(* Logix 5000 AddOnInstructionDefinition export OM_AZ_MOVE; software revision 32.00 *)

ADD_ON_INSTRUCTION OM_AZ_MOVE   (* revision 1.3 U1.0, vendor ORIENTALMOTOR CO.,LTD. *)
// Revision note:
// Implicit message based on AZD-AEP,-CEP and -KEP.
// Help:
// This AOI is used to select and operate a pre-programmed data operation. This is used when the same operation is used repeatedly.
VAR_IN_OUT
   ImplicitMSGinput : INT[28]; {required}   // Implicit message Input (driver->scanner)
        [0]   // Remote I/O (R-OUT)
        [0].0   // R-OUT0
        [0].1   // R-OUT1
        [0].2   // R-OUT2
        [0].3   // R-OUT3
        [0].4   // R-OUT4
        [0].5   // R-OUT5
        [0].6   // R-OUT6
        [0].7   // R-OUT7
        [0].8   // R-OUT8
        [0].9   // R-OUT9
        [0].10   // R-OUT10
        [0].11   // R-OUT11
        [0].12   // R-OUT12
        [0].13   // R-OUT13
        [0].14   // R-OUT14
        [0].15   // R-OUT15
        [1]   // Operation data number selection_R
        [1].0   // M0_R
        [1].1   // M1_R
        [1].2   // M2_R
        [1].3   // M3_R
        [1].4   // M4_R
        [1].5   // M5_R
        [1].6   // M6_R
        [1].7   // M7_R
        [1].8   // Reserved
        [1].9   // Reserved
        [1].10   // Reserved
        [1].11   // Reserved
        [1].12   // Reserved
        [1].13   // Reserved
        [1].14   // Reserved
        [1].15   // Reserved
        [2]   // Fixed I/O (OUT)
        [2].0   // SEQ-BSY
        [2].1   // MOVE
        [2].2   // IN-POS
        [2].3   // START_R
        [2].4   // HOME-END
        [2].5   // READY
        [2].6   // DCMD-RDY
        [2].7   // ALM-A
        [2].8   // TRIG_R
        [2].9   // TRIG-MODE_R
        [2].10   // SET-ERR
        [2].11   // EXE-ERR
        [2].12   // DCMD-FULL
        [2].13   // STOP_R
        [2].14   // ETO-MON
        [2].15   // TLC
        [3]   // Present alarm
        [4]   // Feedback position (lower)
        [5]   // Feedback position (upper)
        [6]   // Feedback speed [Hz] (lower)
        [7]   // Feedback speed [Hz] (upper)
        [8]   // Command position (lower)
        [9]   // Command position (upper)
        [10]   // Torque monitor
        [11]   // CST operating current
        [12]   // Information (lower)
        [13]   // Information (upper)
        [14]   // Reserved
        [15]   // Read parameter ID_R
        [16]   // Read/write status
        [16].0   // Reserved
        [16].1   // Reserved
        [16].2   // Reserved
        [16].3   // Reserved
        [16].4   // Reserved
        [16].5   // Reserved
        [16].6   // Reserved
        [16].7   // RD-ERR
        [16].8   // WR-END
        [16].9   // SYS-BSY
        [16].10   // Reserved
        [16].11   // WR-SET-ERR
        [16].12   // WR-IF-ERR
        [16].13   // WR-NV-ERR
        [16].14   // WR-EXE-ERR
        [16].15   // WR-ERR
        [17]   // Write parameter ID_R
        [18]   // Read data (lower)
        [19]   // Read data (upper)
        [20]   // Assignable monitor 0 (lower)
        [21]   // Assignable monitor 0 (upper)
        [22]   // Assignable monitor 1 (lower)
        [23]   // Assignable monitor 1 (upper)
        [24]   // Assignable monitor 2 (lower)
        [25]   // Assignable monitor 2 (upper)
        [26]   // Assignable monitor 3 (lower)
        [27]   // Assignable monitor 3 (upper)
   ImplicitMSGoutput : INT[20]; {required}   // Implicit message Output (scanner->driver)
        [0]   // Remote I/O(R-IN)
        [0].0   // R-IN0
        [0].1   // R-IN1
        [0].2   // R-IN2
        [0].3   // R-IN3
        [0].4   // R-IN4
        [0].5   // R-IN5
        [0].6   // R-IN6
        [0].7   // R-IN7
        [0].8   // R-IN8
        [0].9   // R-IN9
        [0].10   // R-IN10
        [0].11   // R-IN11
        [0].12   // R-IN12
        [0].13   // R-IN13
        [0].14   // R-IN14
        [0].15   // R-IN15
        [1]   // Operation data number selection
        [1].0   // M0
        [1].1   // M1
        [1].2   // M2
        [1].3   // M3
        [1].4   // M4
        [1].5   // M5
        [1].6   // M6
        [1].7   // M7
        [1].8   // Reserved
        [1].9   // Reserved
        [1].10   // Reserved
        [1].11   // Reserved
        [1].12   // Reserved
        [1].13   // Reserved
        [1].14   // Reserved
        [1].15   // Reserved
        [2]   // Fixed I/O(IN)
        [2].0   // FW-JOG
        [2].1   // RV-JOG
        [2].2   // Reserved
        [2].3   // START
        [2].4   // ZHOME
        [2].5   // STOP
        [2].6   // FREE
        [2].7   // ALM-RST
        [2].8   // TRIG
        [2].9   // TRIG-MODE
        [2].10   // ETO-CLR
        [2].11   // Reserved
        [2].12   // FW-JOG-P
        [2].13   // RV-JOG-P
        [2].14   // FW-POS
        [2].15   // RV-POS
        [3]   // Direct data operation operation type
        [4]   // Direct data operation position (lower)
        [5]   // Direct data operation position (upper)
        [6]   // Direct data operation operating speed (lower)
        [7]   // Direct data operation operating speed (upper)
        [8]   // Direct data operation starting/changing rate (lower)
        [9]   // Direct data operation starting/changing rate (upper)
        [10]   // Direct data operation stopping deceleration (lower)
        [11]   // Direct data operation stopping deceleration (upper)
        [12]   // Direct data operation operating current
        [13]   // Direct data operation forwarding destination
        [14]   // Reserved
        [15]   // Read parameter ID
        [16]   // Write request
        [16].0   // WR-REQ
        [16].1   // Reserved
        [16].2   // Reserved
        [16].3   // Reserved
        [16].4   // Reserved
        [16].5   // Reserved
        [16].6   // Reserved
        [16].7   // Reserved
        [16].8   // Reserved
        [16].9   // Reserved
        [16].10   // Reserved
        [16].11   // Reserved
        [16].12   // Reserved
        [16].13   // Reserved
        [16].14   // Reserved
        [16].15   // Reserved
        [17]   // Write parameter ID
        [18]   // Write data (lower)
        [19]   // Write data (upper)
END_VAR
VAR_INPUT
   Set_Exe : BOOL; {visible}   // Execute AOI
   Set_OpeDataNo : INT; {visible}   // Selected Operation data No.
END_VAR
VAR_OUTPUT
   Sts_Busy : BOOL; {access Read Only, visible}   // Executing status in AOI
   Sts_Err : BOOL; {access Read Only, visible}   // Error status in AOI
   Sts_Done : BOOL; {access Read Only, visible}   // Complete status in AOI
   Read_Present_alarm : INT; {access Read Only, visible}   // Alarm code monitor[Hex]
   Read_Command_position : DINT; {access Read Only, visible}   // Command position monitor[step]
   Read_Feedback_position : DINT; {access Read Only, visible}   // Feedback position monitor[step]
   Read_Torque_monitor : INT; {access Read Only, visible}   // Torque monitor as a percentage of the maximum holding torque(1=0.1%)
   Read_Cumulative_load_monitor : DINT; {access Read Only, visible}   // Cumulative load monitor
END_VAR
VAR
   flag_Exe : BOOL; {access None}
   flag_End : BOOL; {access None}
   flag_Ini : BOOL; {access None}
   flag_Ready : BOOL; {access None}
   flag_Data : BOOL; {access None}
   FixedIO_OUT : INT;   // Fixed I/O(OUT)
        .0   // SEQ-BSY
        .1   // MOVE
        .2   // IN-POS
        .3   // START_R
        .4   // HOME-END
        .5   // READY
        .6   // DCMD-RDY
        .7   // ALM-A
        .8   // TRIG_R
        .9   // TRIG-MODE_R
        .10   // SET-ERR
        .11   // EXE-ERR
        .12   // DCMD-FULL
        .13   // STOP_R
        .14   // ETO-MON
        .15   // TLC
END_VAR

ROUTINE Logic   (* ladder *)
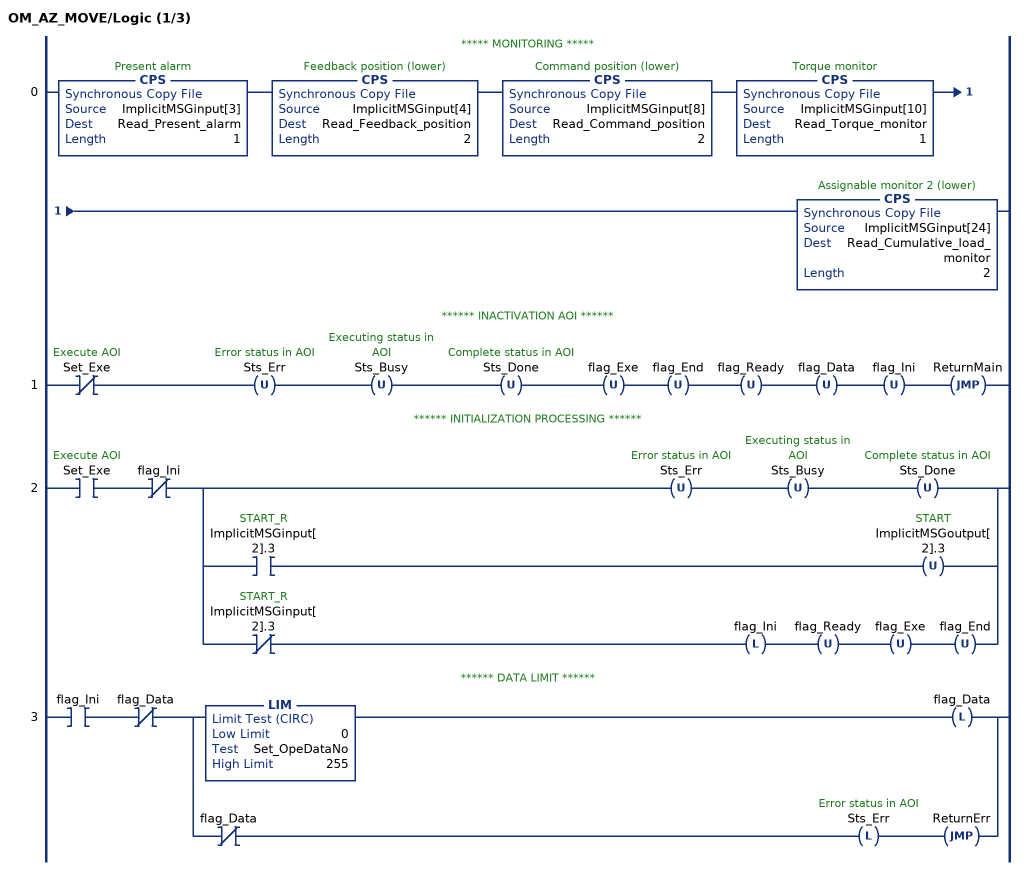
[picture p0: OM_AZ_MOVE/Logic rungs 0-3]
   // ***** MONITORING *****
   0: CPS(ImplicitMSGinput[3],Read_Present_alarm,1)CPS(ImplicitMSGinput[4],Read_Feedback_position,2)CPS(ImplicitMSGinput[8],Read_Command_position,2)CPS(ImplicitMSGinput[10],Read_Torque_monitor,1)CPS(ImplicitMSGinput[24],Read_Cumulative_load_monitor,2);
   // ****** INACTIVATION AOI ******
   1: XIO(Set_Exe)OTU(Sts_Err)OTU(Sts_Busy)OTU(Sts_Done)OTU(flag_Exe)OTU(flag_End)OTU(flag_Ready)OTU(flag_Data)OTU(flag_Ini)JMP(ReturnMain);
   // ****** INITIALIZATION PROCESSING ******
   2: XIC(Set_Exe)XIO(flag_Ini)[OTU(Sts_Err) OTU(Sts_Busy) OTU(Sts_Done) ,[XIC(ImplicitMSGinput[2].3) OTU(ImplicitMSGoutput[2].3) ,XIO(ImplicitMSGinput[2].3) OTL(flag_Ini) OTU(flag_Ready) OTU(flag_Exe) OTU(flag_End) ] ];
   // ****** DATA LIMIT ******
   3: XIC(flag_Ini)XIO(flag_Data)[LIM(0,Set_OpeDataNo,255) OTL(flag_Data) ,XIO(flag_Data) OTL(Sts_Err) JMP(ReturnErr) ];
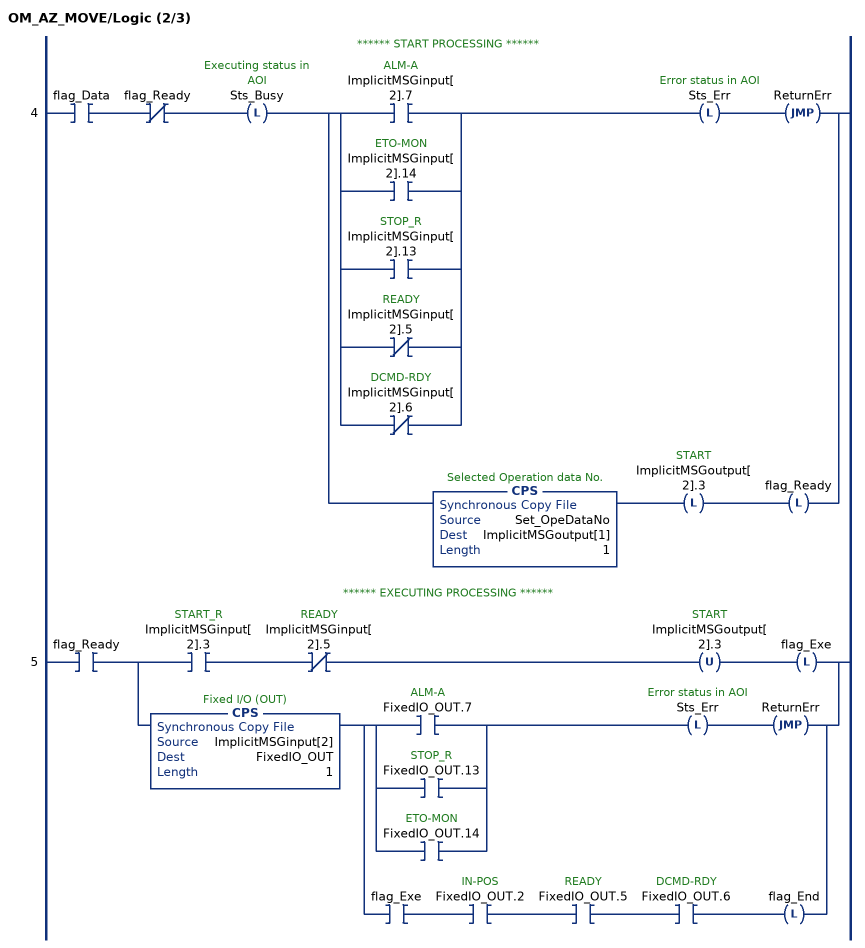
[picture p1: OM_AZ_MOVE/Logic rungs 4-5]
   // ****** START PROCESSING ******
   4: XIC(flag_Data)XIO(flag_Ready)OTL(Sts_Busy)[[XIC(ImplicitMSGinput[2].7) ,XIC(ImplicitMSGinput[2].14) ,XIC(ImplicitMSGinput[2].13) ,XIO(ImplicitMSGinput[2].5) ,XIO(ImplicitMSGinput[2].6) ] OTL(Sts_Err) JMP(ReturnErr) ,CPS(Set_OpeDataNo,ImplicitMSGoutput[1],1) OTL(ImplicitMSGoutput[2].3) OTL(flag_Ready) ];
   // ****** EXECUTING PROCESSING ******
   5: XIC(flag_Ready)[XIC(ImplicitMSGinput[2].3) XIO(ImplicitMSGinput[2].5) OTU(ImplicitMSGoutput[2].3) OTL(flag_Exe) ,CPS(ImplicitMSGinput[2],FixedIO_OUT,1) [[XIC(FixedIO_OUT.7) ,[XIC(FixedIO_OUT.13) ,XIC(FixedIO_OUT.14) ] ] OTL(Sts_Err) JMP(ReturnErr) ,XIC(flag_Exe) XIC(FixedIO_OUT.2) XIC(FixedIO_OUT.5) XIC(FixedIO_OUT.6) OTL(flag_End) ] ];
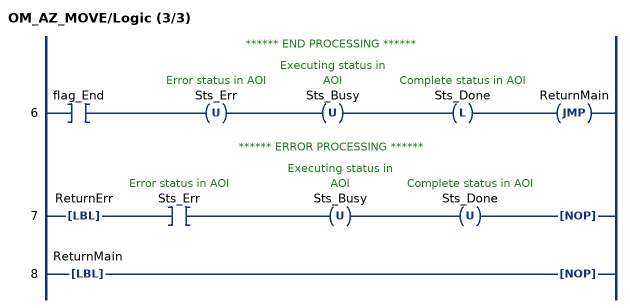
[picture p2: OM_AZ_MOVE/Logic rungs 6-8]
   // ****** END PROCESSING ******
   6: XIC(flag_End)OTU(Sts_Err)OTU(Sts_Busy)OTL(Sts_Done)JMP(ReturnMain);
   // ****** ERROR PROCESSING ******
   7: LBL(ReturnErr)XIC(Sts_Err)OTU(Sts_Busy)OTU(Sts_Done)NOP();
   8: LBL(ReturnMain)NOP();
END_ROUTINE
END_ADD_ON_INSTRUCTION
